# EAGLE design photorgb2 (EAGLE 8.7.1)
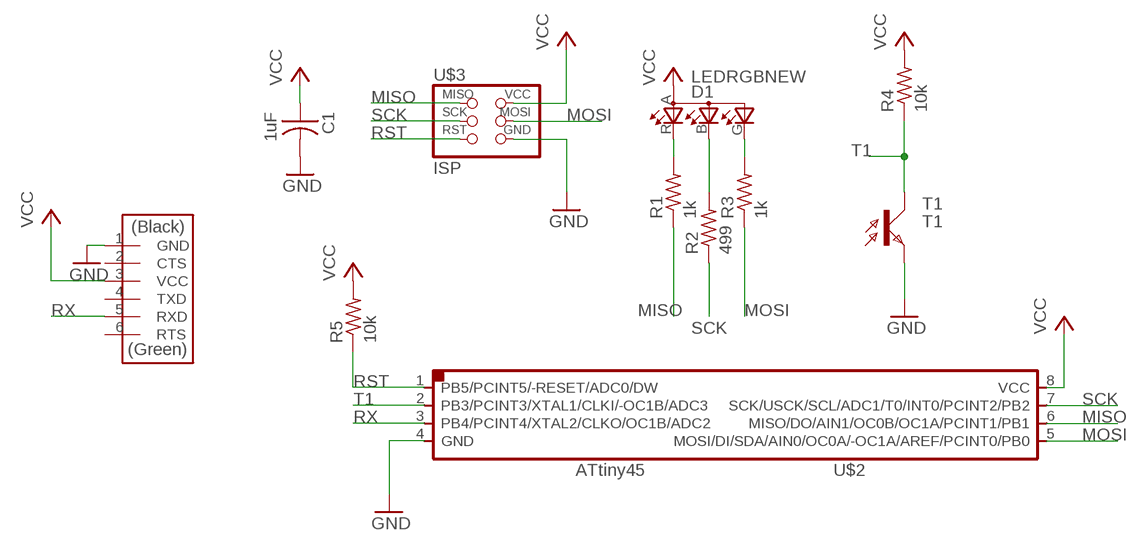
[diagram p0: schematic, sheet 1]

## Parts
C1  1uF  CAP-US1206FAB  [C1206FAB]
D1  LEDRGBNEW  [P-LCC-4]
R1  1k  RES-US1206FAB  [R1206FAB]
R2  499  RES-US1206FAB  [R1206FAB]
R3  1k  RES-US1206FAB  [R1206FAB]
R4  10k  RES-US1206FAB  [R1206FAB]
R5  10k  RES-US1206FAB  [R1206FAB]
T1  T1  PHOTOTRANSISTOR-NPN1206  [OP1206]
U$1  FTDI-SMD-HEADER  [1X06SMD]
U$2  ATTINY45SI  [SOIC8]
U$3  ISP  AVRISPSMD  [2X03SMD]

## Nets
GND: C1.2 T1.EMITTER(E) U$1.1(GND) U$2.4(GND) U$3.6(GND)
MISO: R1.1 U$2.6(MISO/DO/AIN1/OC0B/OC1A/PCINT1/PB1) U$3.1(MISO)
MOSI: R3.1 U$2.5(MOSI/DI/SDA/AIN0/OC0A/-OC1A/AREF/PCINT0/PB0) U$3.4(MOSI)
N$1: D1.R(CRED) R1.2
N$2: D1.G(CGREEN) R3.2
N$3: D1.B(CBLUE) R2.2
RST: R5.1 U$2.1(PB5/PCINT5/-RESET/ADC0/DW) U$3.5(RST)
RX: U$1.5(RXD) U$2.3(PB4/PCINT4/XTAL2/CLKO/OC1B/ADC2)
SCK: R2.1 U$2.7(SCK/USCK/SCL/ADC1/T0/INT0/PCINT2/PB2) U$3.3(SCK)
T1: R4.1 T1.COLLECTOR(C) U$2.2(PB3/PCINT3/XTAL1/CLKI/-OC1B/ADC3)
VCC: C1.1 D1.A(A2) R4.2 R5.2 U$1.3(VCC) U$2.8(VCC) U$3.2(VCC)
Unconnected: U$1.2(CTS) U$1.4(TXD) U$1.6(RTS)

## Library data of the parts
C1 = fab.lbr:CAP-US
D1 = fab.lbr:LEDRGBNEW
R1-R5 = fab.lbr:RES-US: Resistor (US Symbol)
T1 = fab.lbr:PHOTOTRANSISTOR-NPN
U$1 = fab.lbr:FTDI-SMD-HEADER
U$2 = fab.lbr:ATTINY45
U$3 = fab.lbr:AVRISP

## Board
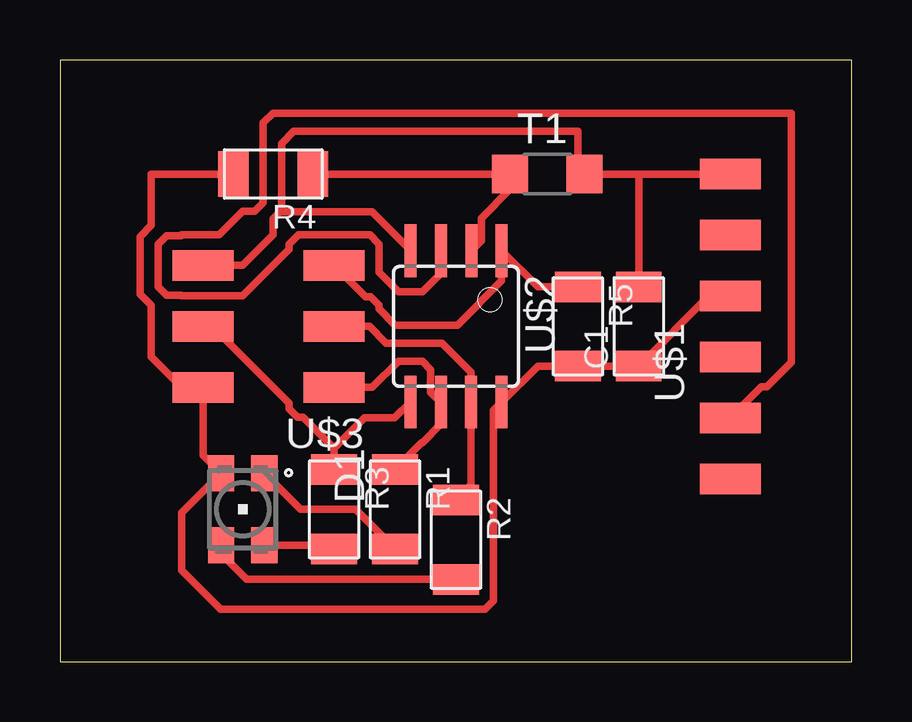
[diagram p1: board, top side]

Size 33 x 25.07 mm. Coordinates in mm from the lower left corner, seen from the top.
Outline: 0,0 33,0 33,25.07 0,25.07 0,0
Copper layers 1: Top 0.035mm
Design rules "basbasic": minimum track width 0.3mm, minimum drill 0.9mm, track to track 0.45mm, track to pad 0.45mm, pad to pad 0.45mm, via to via 0.45mm, smd to smd 6mil, copper to edge 40mil, drill to drill 6mil, minimum pad ring 10mil, minimum via ring 8mil, stop-mask expansion 4mil, vias tented up to drill 0mil, thermal gap 10mil

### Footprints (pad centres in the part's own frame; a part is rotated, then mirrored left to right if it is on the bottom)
C1206FAB = smd 1.27 x 1.905: 1 -1.651,0; 2 1.651,0
P-LCC-4 = smd 1.1 x 1.5: A 0.902,-1.5; B 0.902,1.5; G -0.902,1.5; R -0.902,-1.5
R1206FAB = smd 1.27 x 1.905: 1 -1.651,0; 2 1.651,0
OP1206 = smd 1.5 x 1.6: COLLECTOR -1.55,0; EMITTER 1.55,0
1X06SMD = smd 2.54 x 1.27: 1 0,6.35; 2 0,3.81; 3 0,1.27; 4 0,-1.27; 5 0,-3.81; 6 0,-6.35
SOIC8 = smd 0.5 x 2.2: 1 -1.905,-3.154; 2 -0.645,-3.154; 3 0.625,-3.154; 4 1.895,-3.154; 5 1.905,3.154; 6 0.635,3.154; 7 -0.635,3.154; 8 -1.905,3.154
2X03SMD = smd 2.54 x 1.27: 1 -2.54,2.54; 2 2.92,2.54; 3 -2.54,0; 4 2.92,0; 5 -2.54,-2.54; 6 2.92,-2.54

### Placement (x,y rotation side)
C1  24.13,13.97 90 top
D1  7.62,6.35 180 top
R1  13.97,6.35 270 top
R2  16.51,5.08 270 top
R3  11.43,6.35 270 top
R4  8.89,20.32 180 top
R5  21.59,13.97 270 top
T1  20.32,20.32 0 top
U$1  27.94,13.97 0 top
U$2  16.51,13.97 180 top
U$3  8.89,13.97 180 top

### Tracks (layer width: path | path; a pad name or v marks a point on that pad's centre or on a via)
GND
  Top 0.305: 24.13,20.32 T1.EMITTER 21.59,20.6 21.59,22.1 9.75,22.1 9.23,21.59 9.23,18.8 9.18,18.76 | 24.13,20.32 U$1.1 | 24.13,20.32 C1.2 | U$3.6 7.61,16.51 8.89,17.79 8.89,18.46 9.18,18.76 | 9.18,18.76 13.01,18.76 14.61,17.15 U$2.4
MISO
  Top 0.305: R1.1 15.08,9.11 15.11,9.11 15.87,9.88 U$2.6 15.46,11.23 15.46,12.17 15.11,12.52 14.11,12.52 13.02,11.43 U$3.1
MOSI
  Top 0.305: U$2.5 13.95,10.16 12.7,10.16 11.43,8.89 | 11.43,8.89 R3.1 | U$3.4 6.35,13.97 9.56,10.76 9.56,10.54 9.91,10.19 10.13,10.19 11.43,8.89
N$1
  Top 0.305: R1.2 12.32,6.35 10.02,6.35 D1.R
N$2
  Top 0.305: R3.2 11.28,4.85 D1.G
N$3
  Top 0.305: R2.2 7.79,3.43 6.72,4.5 D1.B
RST
  Top 0.305: R5.1 19.92,15.62 U$2.1 18.42,15.87 16.57,14.03 13.97,14.03 13.3,14.7 13.3,14.85 12.95,15.21 12.73,15.21 U$3.5
RX
  Top 0.305: U$1.5 29.24,11.46 29.46,11.46 30.48,12.48 30.48,22.86 8.89,22.86 8.48,22.45 8.48,19.12 8.12,18.77 7.62,18.77 6.63,17.78 5.08,17.78 5.05,17.75 4.45,17.75 4.1,17.39 4.1,15.62 4.45,15.27 5.05,15.27 5.08,15.24 7.62,15.24 9.56,17.18 9.56,17.39 9.94,17.78 12.92,17.78 13.3,17.39 13.3,16.23 14.11,15.42 15.11,15.42 15.89,16.19 U$2.3
SCK
  Top 0.305: R2.1 17.14,7.37 U$2.7 17.14,12.06 15.94,13.27 13.6,13.27 12.9,13.97 U$3.3
T1
  Top 0.305: R4.1 T1.COLLECTOR 18.77,19.68 17.56,18.47 17.56,17.53 U$2.2
VCC
  Top 0.305: R4.2 3.81,20.32 3.81,18.17 3.34,17.71 3.34,15.31 3.81,14.85 3.81,12.7 5.08,11.43 U$3.2 5.97,8.6 D1.A 5.08,6.21 5.08,3.81 6.7,2.19 17.71,2.19 18.07,2.54 18.07,10.47 U$2.8 19.92,12.32 R5.2 C1.1 27.05,15.24 U$1.3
